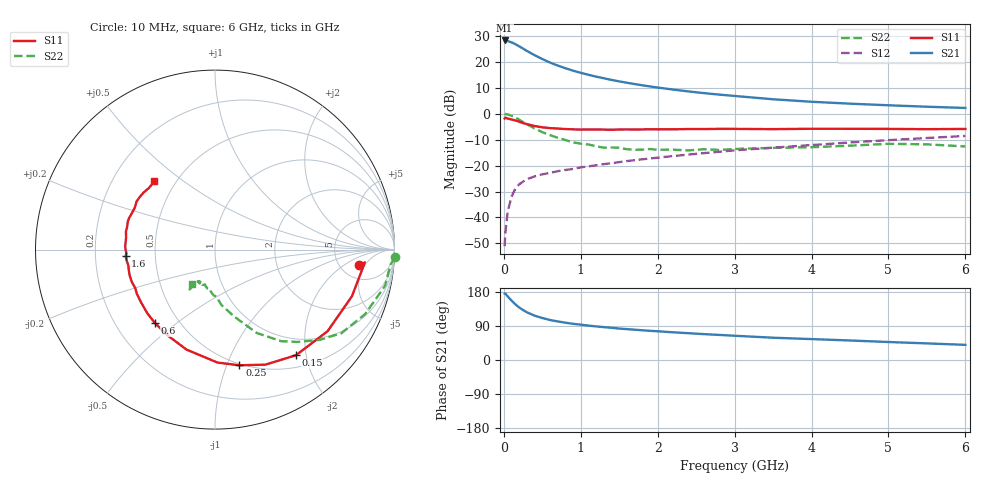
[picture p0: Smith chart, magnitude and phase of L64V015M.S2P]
!  INFINEON TECHNOLOGIES Small Signal Semiconductors
! BFR380L3 , Si-NPN RF-Transistor in TSLP-3-1
!  Vce=4 V,  Ic=15 mA
! Common Emitter S-Parameters:  07. March 2005
#  GHz  S  MA  R  50
! f  S11  S21  S12  S22
! GHz  Mag  Ang  Mag  Ang  Mag  Ang  Mag  Ang
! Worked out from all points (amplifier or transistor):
!   36 points, 10 MHz to 6 GHz, reference 50 ohm
!   highest |S21| = 28.2 dB at 10 MHz (marker M1)
!   |S21| within 3 dB of that: start of sweep to 242.1 MHz
!   unconditionally stable (mu >= 1): 2.24 GHz to 4.733 GHz
!   at 250 MHz: K = 0.29, MSG = 25.6 dB, |S12| = -26.2 dB
!   at 1.4 GHz: K = 0.90, MSG = 16.1 dB, |S12| = -19.1 dB
!   at 6 GHz: K = 0.97, MSG = 5.4 dB, |S12| = -8.6 dB
!   S11 on the Smith chart (normalised r, x): 10 MHz: 7.48, -3.75; 150 MHz: 0.70, -1.82; 250 MHz: 0.49, -1.11; 600 MHz: 0.37, -0.42; 1.6 GHz: 0.33, -0.03; 6 GHz: 0.38, +0.39
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0.01  0.8075 -6.2  25.8 175.6  0.0028 82.6  1.003 -2.5
0.02  0.8382 -4.9  25.63 175.2  0.0051 85.5  0.9812 -4.9
0.05  0.8061 -18.8  25.17 167.8  0.0129 82.8  0.969 -12.0
0.1  0.7749 -35.9  23.7 156.8  0.0253 73.4  0.9109 -23.2
0.15  0.7417 -52.5  21.91 146.8  0.0359 65.5  0.844 -33.5
0.2  0.7 -66.3  19.86 138.5  0.0437 61.7  0.7677 -41.0
0.25  0.6587 -78.1  17.98 131.8  0.0492 57.4  0.689 -48.3
0.3  0.6297 -88.7  16.18 125.9  0.0546 54.9  0.6299 -54.1
0.4  0.5793 -105.9  13.42 117.0  0.062 50.7  0.5192 -63.4
0.5  0.5464 -118.8  11.31 110.8  0.0678 50.3  0.4416 -68.8
0.6  0.5286 -129.3  9.679 105.6  0.0724 49.6  0.3873 -74.1
0.8  0.5062 -144.2  7.533 98.4  0.0823 50.6  0.311 -83.3
0.9  0.5 -150.6  6.746 95.5  0.0862 51.8  0.28 -86.3
1.1  0.4971 -158.9  5.621 90.7  0.0966 53.3  0.255 -91.7
1.4  0.4908 -169.3  4.479 85.0  0.1112 55.6  0.2234 -98.0
1.6  0.499 -175.7  3.947 81.4  0.1223 56.8  0.2068 -105.5
2.2  0.4999 172.2  2.92 73.1  0.1529 59.4  0.2027 -110.8
2.8  0.5105 162.1  2.333 66.2  0.1846 61.0  0.2004 -118.5
3.5  0.5041 152.5  1.897 58.8  0.2215 60.5  0.2195 -120.0
4.5  0.5119 145.5  1.561 51.5  0.279 60.6  0.242 -121.6
5.5  0.5035 137.0  1.363 43.8  0.3404 58.2  0.2566 -122.5
6  0.5088 131.6  1.291 40.0  0.3728 56.5  0.2337 -123.9
